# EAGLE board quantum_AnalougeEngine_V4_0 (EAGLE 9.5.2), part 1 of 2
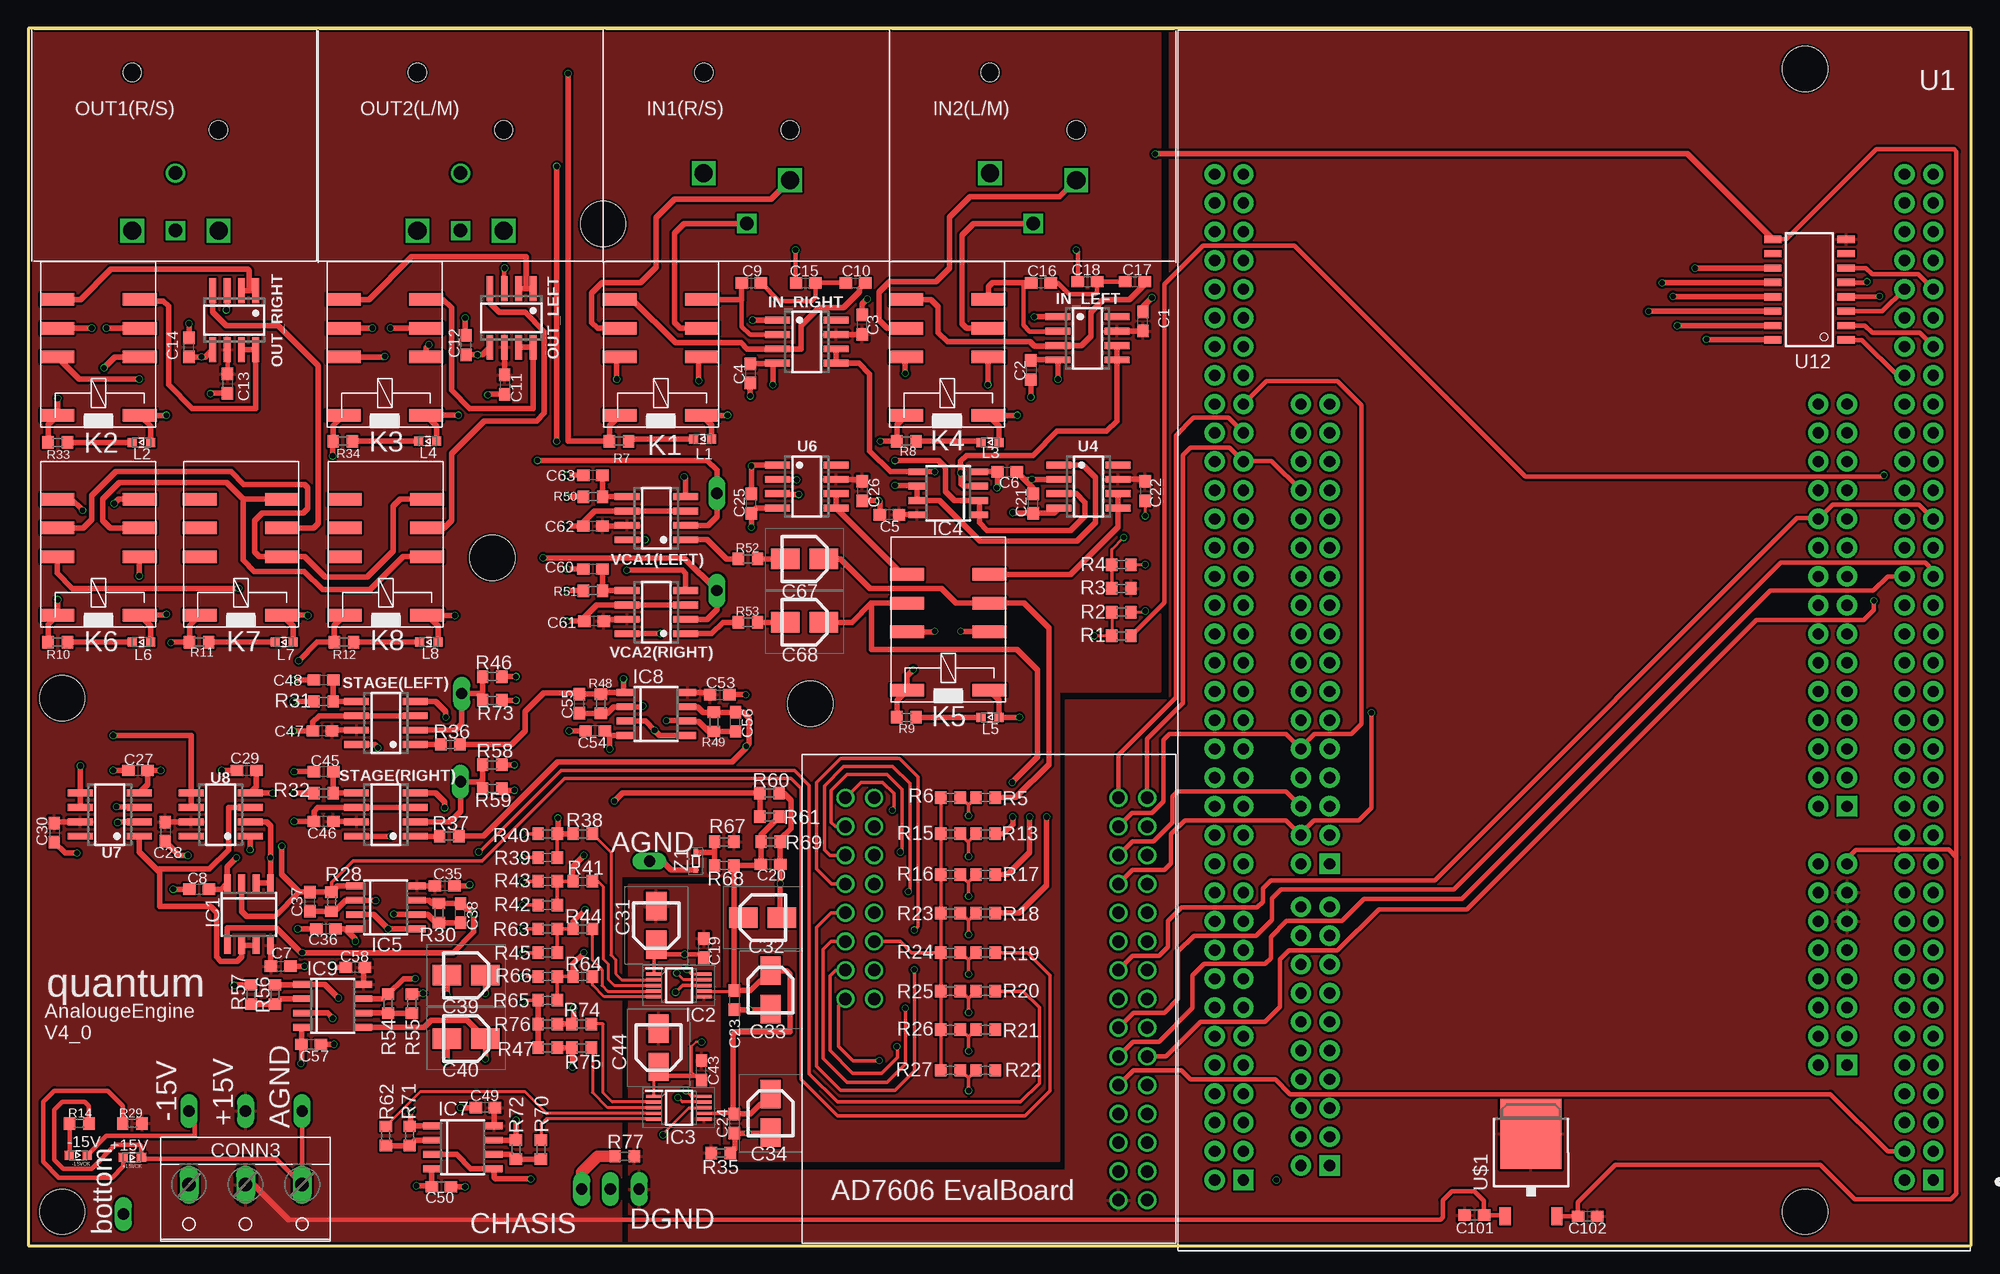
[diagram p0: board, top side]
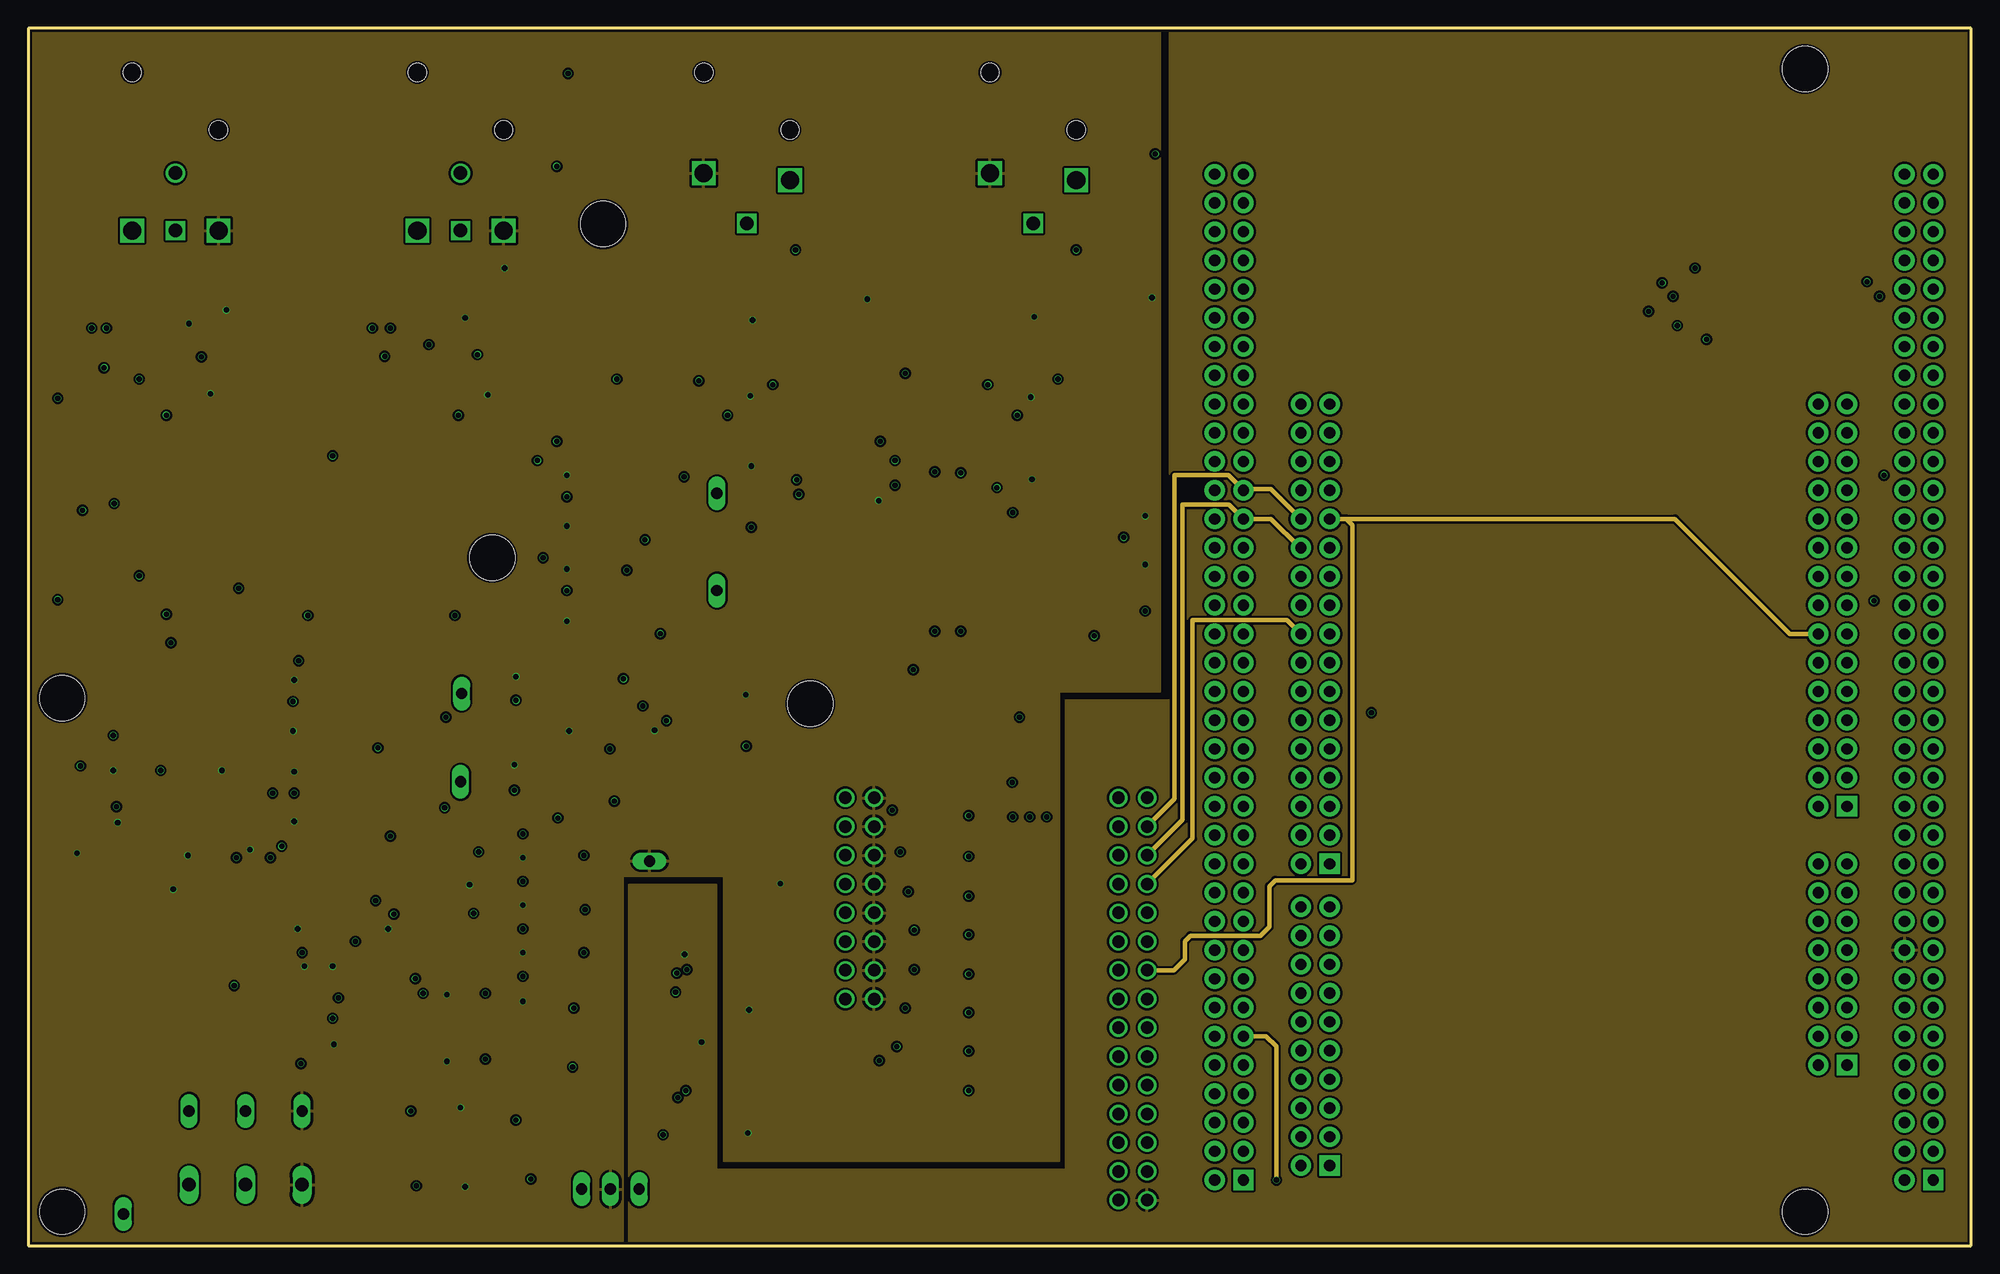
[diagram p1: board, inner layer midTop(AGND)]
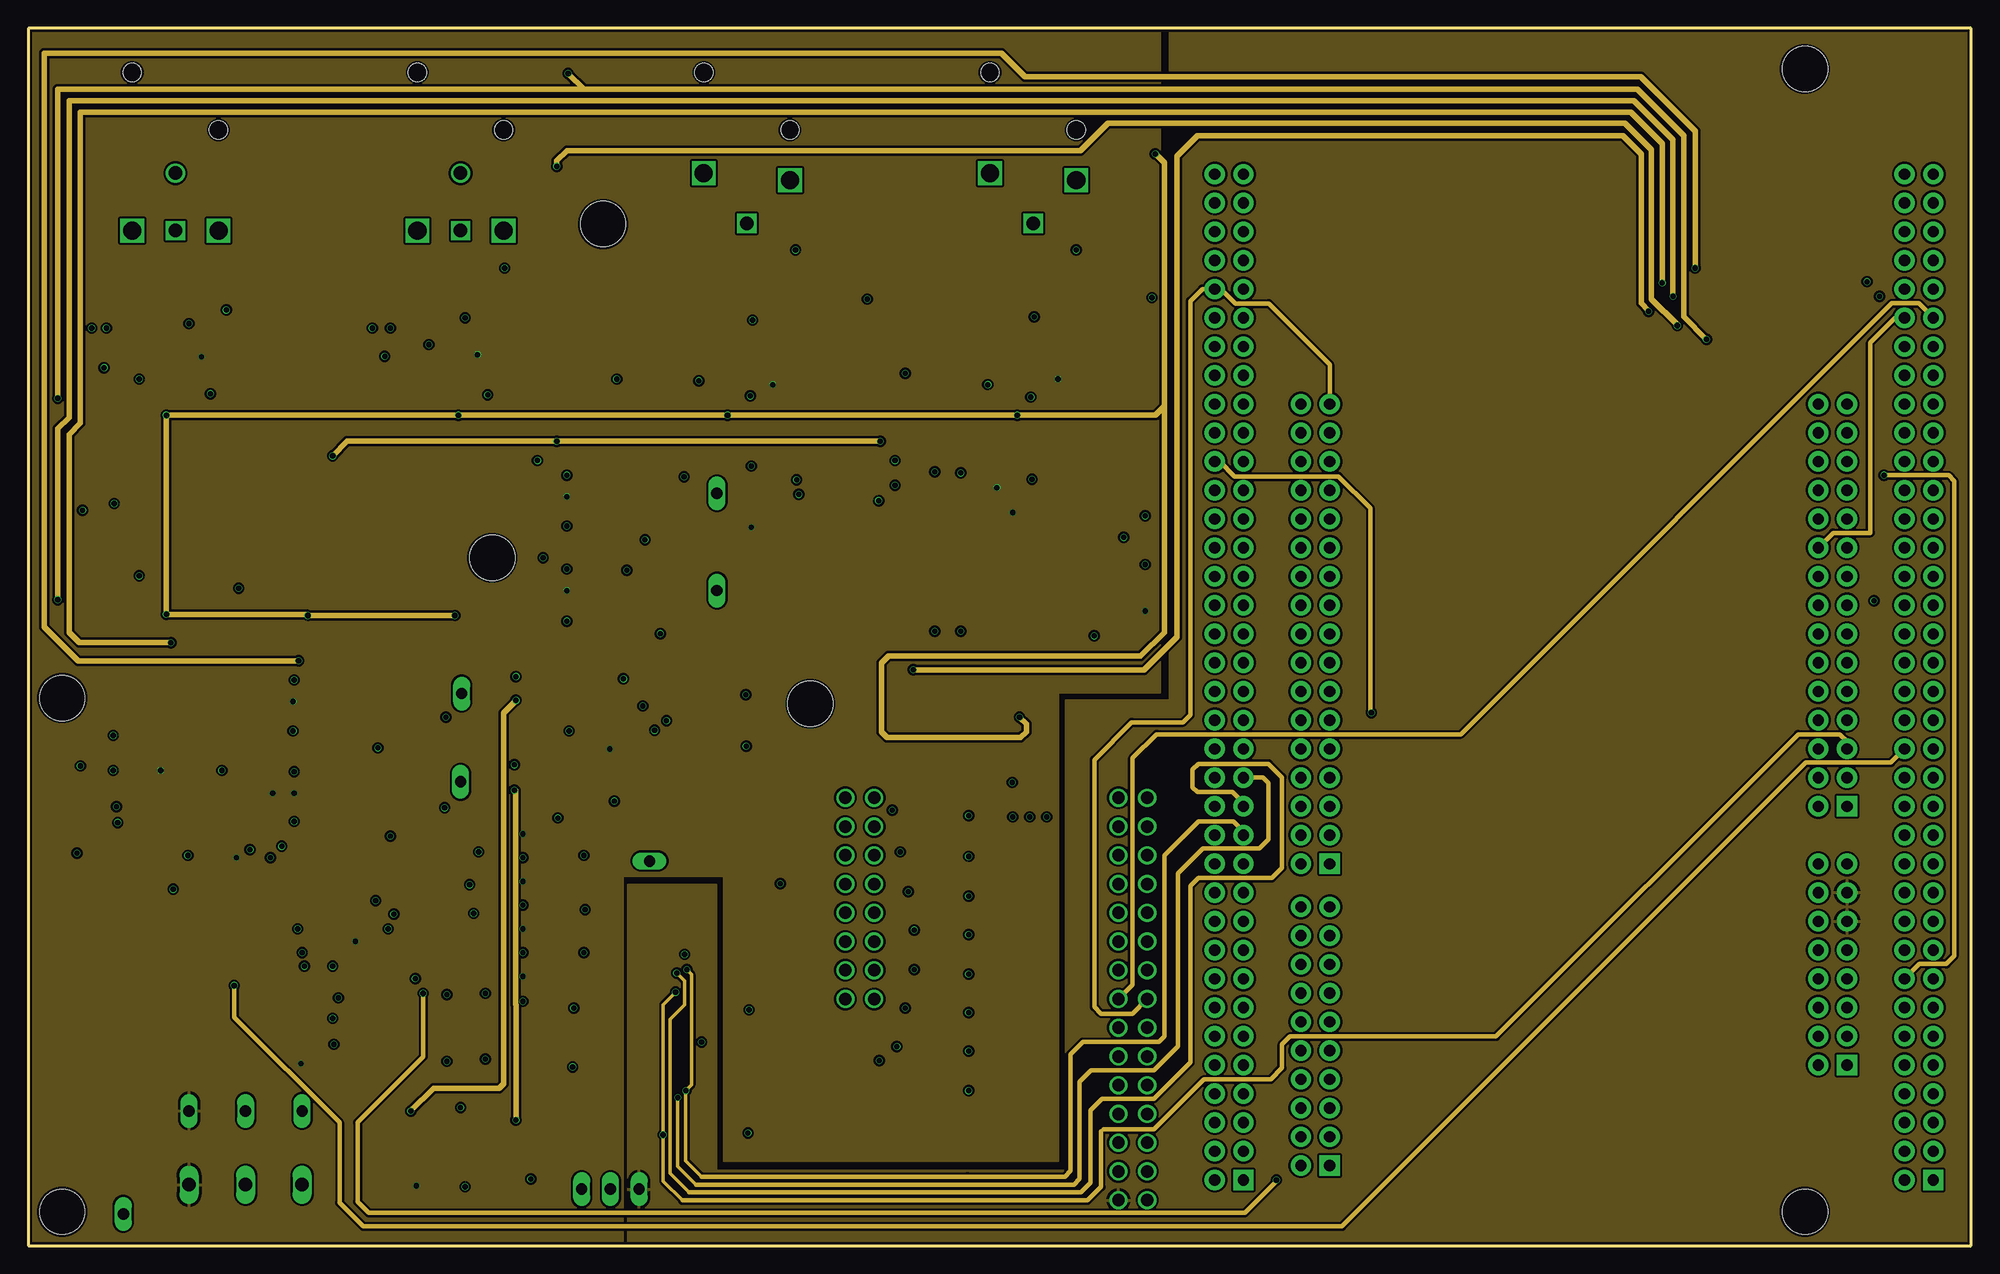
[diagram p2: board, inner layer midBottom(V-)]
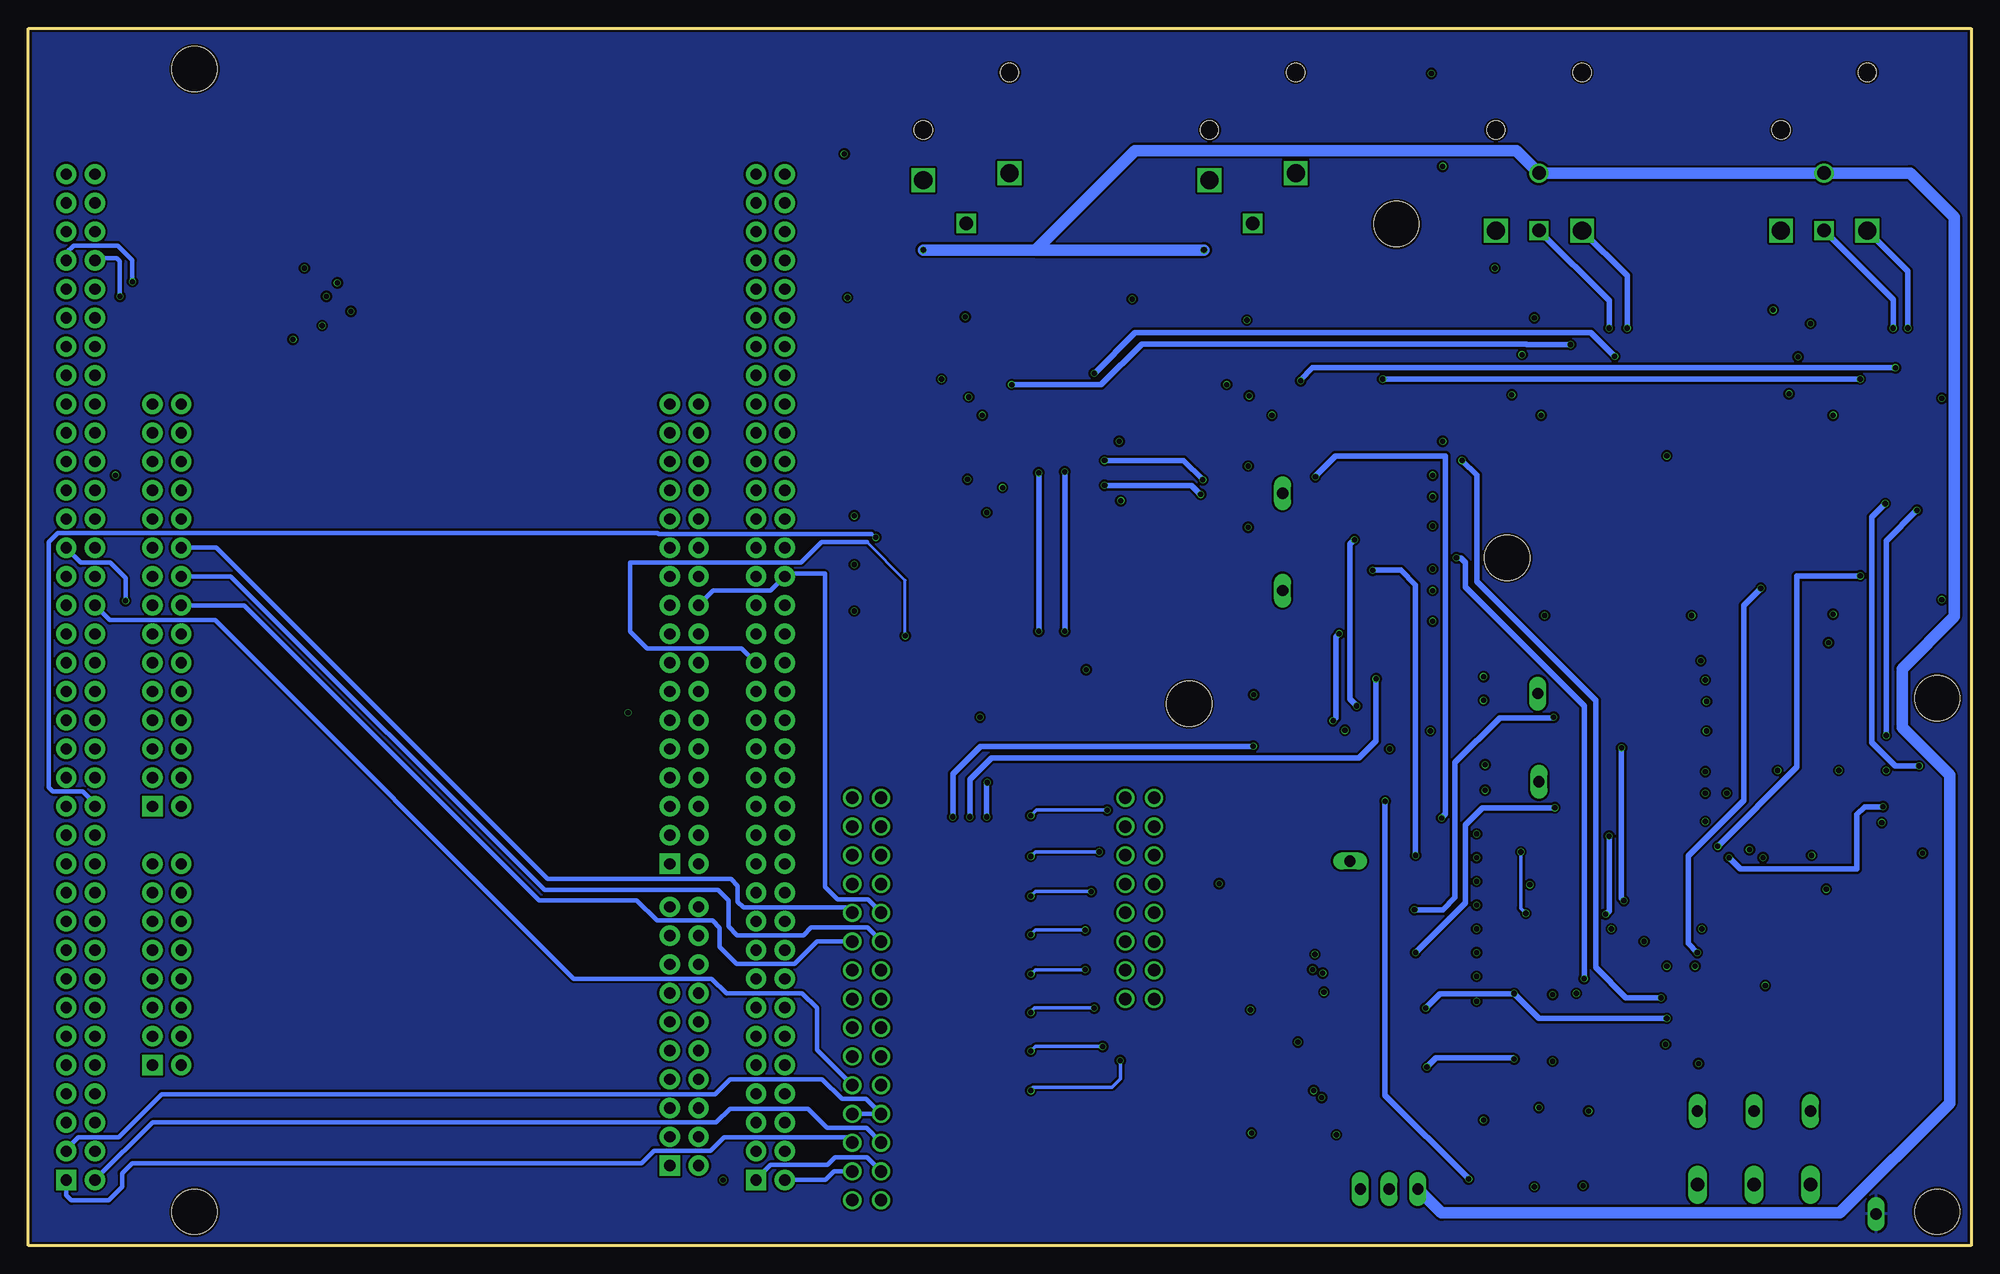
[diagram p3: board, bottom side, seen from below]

Size 171.7 x 107.6 mm. Coordinates in mm from the lower left corner, seen from the top.
Outline: 0,0 171.7,0 171.7,107.6 0,107.6 0,0
Copper layers (1*2+15*16): Top(V+) 0.018mm / dielectric 0.362mm / midTop(AGND) 0.035mm / dielectric 0.71mm / midBottom(V-) 0.035mm / dielectric 0.362mm / Bottom 0.018mm
Design rules "4layer": minimum track width 0.2mm, minimum drill 0.2mm, track to track 0.2mm, track to pad 0.1mm, pad to pad 0.1mm, via to via 0.1mm, smd to smd 0.1mm, copper to edge 0.2mm, drill to drill 0.21mm, minimum pad ring 0.25mm, minimum via ring 0.05mm, stop-mask expansion 0.01mm, vias tented up to drill 0mil, thermal gap 10mil
Holes 4 mm at 3,3 157,3 69.1,47.9 157,104 50.8,90.3 41,60.8 3,48.4

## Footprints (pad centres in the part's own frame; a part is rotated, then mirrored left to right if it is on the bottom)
WL-SMCW_0603 = smd 0.8 x 0.8: 1 -0.8,0; 2 0.8,0
C0603 = smd 1.1 x 1: 1 -0.85,0; 2 0.85,0
CAPAE400X550N = smd 2.5 x 1.8: 1 -1.7,0; 2 1.7,0
W237-103 = drill 1.194 long: 1 -5,-1.29; 2 0,-1.29; 3 5,-1.29
SOIC8 = smd 0.6 x 1.5: 1 -1.905,-2.75; 2 -0.635,-2.75; 3 0.635,-2.75; 4 1.905,-2.75; 5 1.905,2.75; 6 0.635,2.75; 7 -0.635,2.75; 8 -1.905,2.75
SOP50P490X110-10N = smd 1.4 x 0.3: 1 -2.2,1; 2 -2.2,0.5; 3 -2.2,0; 4 -2.2,-0.5; 5 -2.2,-1; 6 2.2,-1; 7 2.2,-0.5; 8 2.2,0; 9 2.2,0.5; 10 2.2,1
NEUTRIK_NC3FAH = drill 1.6 square: 1 -3.81,-12.7; 2 3.81,-13.335 | drill 1.2 square: 3 0,-17.15 | hole 1.6: -3.81,-3.81; 3.81,-8.89
SO08 = smd 0.6 x 2.2: 1 -1.905,-2.6; 2 -0.635,-2.6; 3 0.635,-2.6; 4 1.905,-2.6; 5 1.905,2.6; 6 0.635,2.6; 7 -0.635,2.6; 8 -1.905,2.6
351 = smd 1.11 x 3: 1 -2.623,-3.645; 2 -2.623,3.645; P1 5.096,-3.645; P2 5.096,3.645; Q1 2.556,-3.645; Q2 2.556,3.645; S1 7.636,-3.645; S2 7.636,3.645
NEUTRIK_NC3MAH = drill 1.6 square: 1 3.81,-17.78; 2 -3.81,-17.78 | drill 1.2 square: 3 0,-17.78 | drill 1.2: G 0,-12.7 | hole 1.6: -3.81,-3.8; 3.81,-8.89
R0603 = smd 1 x 1.1: 1 -0.85,0; 2 0.85,0
THT_PIN = drill 1 long: P$1 0,0
MODULE_NUCLEO-F429ZI = drill 1 pad 1.8 square: CN7_1 21.59,43.82; CN8_1 -24.13,34.93; CN9_1 -24.13,12.07; CN10_1 21.59,17.15; CN11_1 -31.75,45.09; CN12_1 29.21,45.09 | drill 1 pad 1.8: CN7_2 24.13,43.82; CN7_3 21.59,41.28; CN7_4 24.13,41.28; CN7_5 21.59,38.74; CN7_6 24.13,38.74; CN7_7 21.59,36.2; CN7_8 24.13,36.2; CN7_9 21.59,33.66; CN7_10 24.13,33.66; CN7_11 21.59,31.12; CN7_12 24.13,31.12; CN7_13 21.59,28.58; CN7_14 24.13,28.58; CN7_15 21.59,26.04; CN7_16 24.13,26.04; CN7_17 21.59,23.5; CN7_18 24.13,23.5; CN7_19 21.59,20.96; CN7_20 24.13,20.96; CN8_2 -21.59,34.93; CN8_3 -24.13,32.39; CN8_4 -21.59,32.39; CN8_5 -24.13,29.85; CN8_6 -21.59,29.85; CN8_7 -24.13,27.31; CN8_8 -21.59,27.31; CN8_9 -24.13,24.77; CN8_10 -21.59,24.77; CN8_11 -24.13,22.23; CN8_12 -21.59,22.23; CN8_13 -24.13,19.69; CN8_14 -21.59,19.69; CN8_15 -24.13,17.15; CN8_16 -21.59,17.15; CN9_2 -21.59,12.07; CN9_3 -24.13,9.53; CN9_4 -21.59,9.53; CN9_5 -24.13,6.99; CN9_6 -21.59,6.99; CN9_7 -24.13,4.45; CN9_8 -21.59,4.45; CN9_9 -24.13,1.91; CN9_10 -21.59,1.91; CN9_11 -24.13,-0.63; CN9_12 -21.59,-0.63; CN9_13 -24.13,-3.17; CN9_14 -21.59,-3.17; CN9_15 -24.13,-5.71; CN9_16 -21.59,-5.71; CN9_17 -24.13,-8.25; CN9_18 -21.59,-8.25; CN9_19 -24.13,-10.79; CN9_20 -21.59,-10.79; CN9_21 -24.13,-13.33; CN9_22 -21.59,-13.33; CN9_23 -24.13,-15.87; CN9_24 -21.59,-15.87; CN9_25 -24.13,-18.41; CN9_26 -21.59,-18.41; CN9_27 -24.13,-20.95; CN9_28 -21.59,-20.95; CN9_29 -24.13,-23.49; CN9_30 -21.59,-23.49; CN10_2 24.13,17.15; CN10_3 21.59,14.61; CN10_4 24.13,14.61; CN10_5 21.59,12.07; CN10_6 24.13,12.07; CN10_7 21.59,9.53; CN10_8 24.13,9.53; CN10_9 21.59,6.99; CN10_10 24.13,6.99; CN10_11 21.59,4.45; CN10_12 24.13,4.45; CN10_13 21.59,1.91; CN10_14 24.13,1.91; CN10_15 21.59,-0.63; CN10_16 24.13,-0.63; CN10_17 21.59,-3.17; CN10_18 24.13,-3.17; CN10_19 21.59,-5.71; CN10_20 24.13,-5.71; CN10_21 21.59,-8.25; CN10_22 24.13,-8.25; CN10_23 21.59,-10.79; CN10_24 24.13,-10.79; CN10_25 21.59,-13.33; CN10_26 24.13,-13.33; CN10_27 21.59,-15.87; CN10_28 24.13,-15.87; CN10_29 21.59,-18.41; CN10_30 24.13,-18.41; CN10_31 21.59,-20.95; CN10_32 24.13,-20.95; CN10_33 21.59,-23.49; CN10_34 24.13,-23.49; CN11_2 -29.21,45.09; CN11_3 -31.75,42.55; CN11_4 -29.21,42.55; CN11_5 -31.75,40.01; CN11_6 -29.21,40.01; CN11_7 -31.75,37.47; CN11_8 -29.21,37.47; CN11_9 -31.75,34.93; CN11_10 -29.21,34.93; CN11_11 -31.75,32.39; CN11_12 -29.21,32.39; CN11_13 -31.75,29.85; CN11_14 -29.21,29.85; CN11_15 -31.75,27.31; CN11_16 -29.21,27.31; CN11_17 -31.75,24.77; CN11_18 -29.21,24.77; CN11_19 -31.75,22.23; CN11_20 -29.21,22.23; CN11_21 -31.75,19.69; CN11_22 -29.21,19.69; CN11_23 -31.75,17.15; CN11_24 -29.21,17.15; CN11_25 -31.75,14.61; CN11_26 -29.21,14.61; CN11_27 -31.75,12.07; CN11_28 -29.21,12.07; CN11_29 -31.75,9.53; CN11_30 -29.21,9.53; CN11_31 -31.75,6.99; CN11_32 -29.21,6.99; CN11_33 -31.75,4.45; CN11_34 -29.21,4.45; CN11_35 -31.75,1.91; CN11_36 -29.21,1.91; CN11_37 -31.75,-0.63; CN11_38 -29.21,-0.63; CN11_39 -31.75,-3.17; CN11_40 -29.21,-3.17; CN11_41 -31.75,-5.71; CN11_42 -29.21,-5.71; CN11_43 -31.75,-8.25; CN11_44 -29.21,-8.25; CN11_45 -31.75,-10.79; CN11_46 -29.21,-10.79; CN11_47 -31.75,-13.33; CN11_48 -29.21,-13.33; CN11_49 -31.75,-15.87; CN11_50 -29.21,-15.87; CN11_51 -31.75,-18.41; CN11_52 -29.21,-18.41; CN11_53 -31.75,-20.95; CN11_54 -29.21,-20.95; CN11_55 -31.75,-23.49; CN11_56 -29.21,-23.49; CN11_57 -31.75,-26.03; CN11_58 -29.21,-26.03; CN11_59 -31.75,-28.57; CN11_60 -29.21,-28.57; CN11_61 -31.75,-31.11; CN11_62 -29.21,-31.11; CN11_63 -31.75,-33.65; CN11_64 -29.21,-33.65; CN11_65 -31.75,-36.19; CN11_66 -29.21,-36.19; CN11_67 -31.75,-38.73; CN11_68 -29.21,-38.73; CN11_69 -31.75,-41.27; CN11_70 -29.21,-41.27; CN11_71 -31.75,-43.81; CN11_72 -29.21,-43.81; CN12_2 31.75,45.09; CN12_3 29.21,42.55; CN12_4 31.75,42.55; CN12_5 29.21,40.01; CN12_6 31.75,40.01; CN12_7 29.21,37.47; CN12_8 31.75,37.47; CN12_9 29.21,34.93; CN12_10 31.75,34.93; CN12_11 29.21,32.39; CN12_12 31.75,32.39; CN12_13 29.21,29.85; CN12_14 31.75,29.85; CN12_15 29.21,27.31; CN12_16 31.75,27.31; CN12_17 29.21,24.77; CN12_18 31.75,24.77; CN12_19 29.21,22.23; CN12_20 31.75,22.23; CN12_21 29.21,19.69; CN12_22 31.75,19.69; CN12_23 29.21,17.15; CN12_24 31.75,17.15; CN12_25 29.21,14.61; CN12_26 31.75,14.61; CN12_27 29.21,12.07; CN12_28 31.75,12.07; CN12_29 29.21,9.53; CN12_30 31.75,9.53; CN12_31 29.21,6.99; CN12_32 31.75,6.99; CN12_33 29.21,4.45; CN12_34 31.75,4.45; CN12_35 29.21,1.91; CN12_36 31.75,1.91; CN12_37 29.21,-0.63; CN12_38 31.75,-0.63; CN12_39 29.21,-3.17; CN12_40 31.75,-3.17; CN12_41 29.21,-5.71; CN12_42 31.75,-5.71; CN12_43 29.21,-8.25; CN12_44 31.75,-8.25; CN12_45 29.21,-10.79; CN12_46 31.75,-10.79; CN12_47 29.21,-13.33; CN12_48 31.75,-13.33; CN12_49 29.21,-15.87; CN12_50 31.75,-15.87; CN12_51 29.21,-18.41; CN12_52 31.75,-18.41; CN12_53 29.21,-20.95; CN12_54 31.75,-20.95; CN12_55 29.21,-23.49; CN12_56 31.75,-23.49; CN12_57 29.21,-26.03; CN12_58 31.75,-26.03; CN12_59 29.21,-28.57; CN12_60 31.75,-28.57; CN12_61 29.21,-31.11; CN12_62 31.75,-31.11; CN12_63 29.21,-33.65; CN12_64 31.75,-33.65; CN12_65 29.21,-36.19; CN12_66 31.75,-36.19; CN12_67 29.21,-38.73; CN12_68 31.75,-38.73; CN12_69 29.21,-41.27; CN12_70 31.75,-41.27; CN12_71 29.21,-43.81; CN12_72 31.75,-43.81
SOIC16 = smd 1.524 x 0.635: 1 -3.24,4.445; 2 -3.24,3.175; 3 -3.24,1.905; 4 -3.24,0.635; 5 -3.24,-0.635; 6 -3.24,-1.905; 7 -3.24,-3.175; 8 -3.24,-4.445; 9 3.24,-4.445; 10 3.24,-3.175; 11 3.24,-1.905; 12 3.24,-0.635; 13 3.24,0.635; 14 3.24,1.905; 15 3.24,3.175; 16 3.24,4.445
TO252 = smd 1 x 1.6: 1 -2.28,-4.8; 3 2.28,-4.8 | smd 5.4 x 6.2: 2 0,2.5
AD7606_EVALBOARD = drill 1.1: +5V 30.48,-39.37; BUSY 27.94,-26.67; CS 30.48,-26.67; CVA 30.48,-31.75; CVB 27.94,-31.75; DB0 30.48,-21.59; DB1 27.94,-21.59; DB2 30.48,-19.05; DB3 27.94,-19.05; DB4 30.48,-16.51; DB5 27.94,-16.51; DB6 30.48,-13.97; DB7 27.94,-13.97; DB8 30.48,-11.43; DB9 27.94,-11.43; DB10 30.48,-8.89; DB11 27.94,-8.89; DB12 30.48,-6.35; DB13 27.94,-6.35; DB14 30.48,-3.81; DB15 27.94,-3.81; FRST 27.94,-24.13; G1 6.35,-3.81; G2 6.35,-6.35; G3 6.35,-8.89; G4 6.35,-11.43; G5 6.35,-13.97; G6 6.35,-16.51; G7 6.35,-19.05; G8 6.35,-21.59; GND 27.94,-39.37; OS0 30.48,-36.83; OS1 27.94,-36.83; OS2 30.48,-34.29; RANGE 27.94,-34.29; RD 27.94,-29.21; RST 30.48,-29.21; V1 3.81,-3.81; V2 3.81,-6.35; V3 3.81,-8.89; V4 3.81,-11.43; V5 3.81,-13.97; V6 3.81,-16.51; V7 3.81,-19.05; V8 3.81,-21.59; VIO 30.48,-24.13
SODFL1608X65N = smd 0.57 x 0.42: 1 -0.775,0; 2 0.775,0

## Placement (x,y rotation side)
+15VOK  SMD_LED_0603  [WL-SMCW_0603]  9.2,7.8 180 top
-15VOK  SMD_LED_0603  [WL-SMCW_0603]  4.4,8 180 top
C1  100nF  [C0603]  98.5,81.7 90 top
C2  100nF  [C0603]  88.6,77.4 270 top
C3  100nF  [C0603]  73.7,81.4 90 top
C4  100nF  [C0603]  63.8,77.1 270 top
C5  100nF  [C0603]  76.1,64.6 180 top
C6  100nF  [C0603]  86.5,68.4 0 top
C7  100nF  [C0603]  22.3,24.7 0 top
C8  100nF  [C0603]  15.1,31.5 180 top
C9  470 pF  [C0603]  63.9,85.1 0 top
C10  470 pF  [C0603]  73.1,85.1 0 top
C11  100nF  [C0603]  42.1,76.1 270 top
C12  100nF  [C0603]  38.7,79.6 90 top
C13  100nF  [C0603]  17.6,76.2 270 top
C14  100nF  [C0603]  14.2,79.4 90 top
C15  47 pF  [C0603]  68.7,85.1 0 top
C16  470 pF  [C0603]  89.5,85.1 0 top
C17  470 pF  [C0603]  97.8,85.2 0 top
C18  47 pF  [C0603]  93.6,85.2 0 top
C19  100nF  [C0603]  59.7,26.3 90 top
C20  100nF  [C0603]  65.6,33.7 0 top
C21  100nF  [C0603]  88.8,65.6 90 top
C22  100nF  [C0603]  98.7,66.7 270 top
C23  100nF  [C0603]  62.4,21.7 270 top
C24  100nF  [C0603]  62.4,10.8 270 top
C25  100nF  [C0603]  63.9,65.6 90 top
C26  100nF  [C0603]  73.7,66.7 270 top
C27  100nF  [C0603]  9.7,42 180 top
C28  100nF  [C0603]  12.1,36.6 270 top
C29  100nF  [C0603]  19.3,42 180 top
C30  100nF  [C0603]  2.3,36.5 270 top
C31  10 µF  [CAPAE400X550N]  55.5,28.3 90 top
C32  10 µF  [CAPAE400X550N]  64.9,29 0 top
C33  10 µF  [CAPAE400X550N]  65.6,22.6 270 top
C34  10 µF  [CAPAE400X550N]  65.6,11.7 270 top
C35  100nF  [C0603]  36.8,31.8 0 top
C36  100nF  [C0603]  26.3,28 180 top
C37  22pF  [C0603]  24.9,30.4 90 top
C38  22pF  [C0603]  38.2,29.4 90 top
C39  10 µF  [CAPAE400X550N]  38.7,23.9 180 top
C40  10 µF  [CAPAE400X550N]  38.7,18.3 180 top
C43  100nF  [C0603]  59.5,15.5 90 top
C44  10 µF  [CAPAE400X550N]  55.7,17.5 90 top
C45  100nF  [C0603]  26.1,41.9 180 top
C46  100nF  [C0603]  26.1,37.5 180 top
C47  100nF  [C0603]  26,45.5 180 top
C48  100nF  [C0603]  26.1,50 180 top
C49  100nF  [C0603]  40.4,12.2 180 top
C50  100nF  [C0603]  36.5,5.2 0 top
C53  100nF  [C0603]  61.1,48.7 0 top
C54  100nF  [C0603]  50.1,45.5 180 top
C55  22pF  [C0603]  48.7,47.9 90 top
C56  22pF  [C0603]  62.5,46.3 90 top
C57  100nF  [C0603]  25,17.8 0 top
C58  100nF  [C0603]  28.9,24.6 180 top
C60  100nF  [C0603]  49.9,59.8 180 top
C61  100nF  [C0603]  50,55.2 180 top
C62  100nF  [C0603]  49.9,63.6 180 top
C63  100nF  [C0603]  49.9,68.1 180 top
C67  47µF  [CAPAE400X550N]  68.6,60.7 180 top
C68  47µF  [CAPAE400X550N]  68.6,55.1 180 top
C101  [C0603]  127.8,2.7 180 top
C102  [C0603]  137.8,2.6 0 top
CONN3  [W237-103]  19.2,4.1 180 top
IC1  OP275  [SOIC8]  19.5,29.3 180 top
IC2  DAC084S085CIMM_NOPB  [SOP50P490X110-10N]  57.5,23 0 top
IC3  DAC084S085CIMM_NOPB  [SOP50P490X110-10N]  57.5,12.2 0 top
IC4  OP275  [SOIC8]  81.3,66.5 90 top
IC5  OP275  [SOIC8]  31.6,29.9 270 top
IC7  TL072  [SOIC8]  38.4,8.7 270 top
IC8  OP275  [SOIC8]  55.5,47 270 top
IC9  TL072  [SOIC8]  26.9,21.2 270 top
IN1(R/S)  NEUTRIK_NC3FAH  [NEUTRIK_NC3FAH]  63.5,107.5 0 top
IN2(L/M)  NEUTRIK_NC3FAH  [NEUTRIK_NC3FAH]  88.8,107.5 0 top
IN_LEFT  1240  [SO08]  93.6,80.2 270 top
IN_RIGHT  1240  [SO08]  68.8,79.9 270 top
K1  K1  [351]  55.9,76 90 top
K2  K2  [351]  6.2,76 90 top
K3  K3  [351]  31.5,76 90 top
K4  K4  [351]  81.2,76 90 top
K5  RELAY_EE2-5NU  [351]  81.3,51.7 90 top
K6  RELAY_EE2-5NU  [351]  6.2,58.35 90 top
K7  RELAY_EE2-5NU  [351]  18.8,58.35 90 top
K8  RELAY_EE2-5NU  [351]  31.6,58.35 90 top
L1  SMD_LED_0603  [WL-SMCW_0603]  59.6,71.3 0 top
L2  SMD_LED_0603  [WL-SMCW_0603]  10,71 0 top
L3  SMD_LED_0603  [WL-SMCW_0603]  85,71 0 top
L4  SMD_LED_0603  [WL-SMCW_0603]  35.3,71.1 0 top
L5  SMD_LED_0603  [WL-SMCW_0603]  85,46.7 0 top
L6  SMD_LED_0603  [WL-SMCW_0603]  10,53.35 0 top
L7  SMD_LED_0603  [WL-SMCW_0603]  22.6,53.35 0 top
L8  SMD_LED_0603  [WL-SMCW_0603]  35.4,53.35 0 top
OUT1(R/S)  NEUTRIK_NC3MAH  [NEUTRIK_NC3MAH]  13,107.5 0 top
OUT2(L/M)  NEUTRIK_NC3MAH  [NEUTRIK_NC3MAH]  38.2,107.5 0 top
OUT_LEFT  1646  [SO08]  42.7,82 180 top
OUT_RIGHT  1646  [SO08]  18.2,81.8 180 top
R1  10k  [R0603]  96.6,53.9 0 top
R2  100k  [R0603]  96.6,56 180 top
R3  100k  [R0603]  96.6,58.1 0 top
R4  10k  [R0603]  96.6,60.2 180 top
R5  10k  [R0603]  84.6,39.6 180 top
R6  10k  [R0603]  81.5,39.6 0 top
R7  500R  [R0603]  52.2,71.1 0 top
R8  500R  [R0603]  77.6,71.1 0 top
R9  500R  [R0603]  77.6,46.7 0 top
R10  500R  [R0603]  2.6,53.35 0 top
R11  500R  [R0603]  15.1,53.35 0 top
R12  500R  [R0603]  27.9,53.35 0 top
R13  10k  [R0603]  84.6,36.4 180 top
R14  220R  [R0603]  4.5,10.8 0 top
R15  10k  [R0603]  81.5,36.4 0 top
R16  10k  [R0603]  81.5,32.8 0 top
R17  10k  [R0603]  84.6,32.8 180 top
R18  10k  [R0603]  84.6,29.4 180 top
R19  10k  [R0603]  84.6,25.9 180 top
R20  10k  [R0603]  84.6,22.5 180 top
R21  10k  [R0603]  84.6,19.1 180 top
R22  10k  [R0603]  84.6,15.5 180 top
R23  10k  [R0603]  81.5,29.4 0 top
R24  10k  [R0603]  81.5,25.9 0 top
R25  10k  [R0603]  81.5,22.5 0 top
R26  10k  [R0603]  81.5,19.1 0 top
R27  10k  [R0603]  81.5,15.5 0 top
R28  20k  [R0603]  26.8,30.4 90 top
R29  220R  [R0603]  9.2,10.8 0 top
R30  20k  [R0603]  36.3,29.4 90 top
R31  5k1  [R0603]  26.1,48.1 0 top
R32  5k1  [R0603]  26.1,40 0 top
R33  500R  [R0603]  2.6,71 0 top
R34  500R  [R0603]  27.8,71.1 0 top
R35  0R  [R0603]  61.2,8.2 180 top
R36  20k  [R0603]  37.3,44.3 180 top
R37  20k  [R0603]  37.2,36.2 180 top
R38  51k  [R0603]  49,36.4 0 top
R39  51R  [R0603]  45.9,34.3 0 top
R40  90k9  [R0603]  45.9,36.4 0 top
R41  51k  [R0603]  49,32.2 0 top
R42  51R  [R0603]  45.9,30.1 0 top
R43  90k9  [R0603]  45.9,32.2 0 top
R44  51k  [R0603]  49,28 0 top
R45  51R  [R0603]  45.9,25.9 0 top
R46  10k  [R0603]  41,50.3 180 top
R47  1k8  [R0603]  45.9,17.5 0 top
R48  20k  [R0603]  50.6,47.9 90 top
R49  20k  [R0603]  60.6,46.3 90 top
R50  5k1  [R0603]  49.9,66.2 0 top
R51  5k1  [R0603]  49.9,57.9 0 top
R52  20k  [R0603]  63.6,60.7 180 top
R53  20k  [R0603]  63.6,55.1 180 top
R54  10k  [R0603]  31.8,21.4 90 top
R55  10k  [R0603]  33.9,21.4 270 top
R56  10k  [R0603]  21.8,22.2 90 top
R57  10k  [R0603]  19.7,22.2 270 top
R58  10k  [R0603]  41,42.5 180 top
R59  56k  [R0603]  41,40.4 0 top
R60  10k  [R0603]  65.5,40 180 top
R61  10k  [R0603]  65.5,37.9 0 top
R62  10k  [R0603]  31.6,9.7 270 top
R63  90k9  [R0603]  45.9,28 0 top
R64  51k  [R0603]  49,23.8 0 top
R65  51R  [R0603]  45.9,21.7 0 top
R66  90k9  [R0603]  45.9,23.8 0 top
R67  10k  [R0603]  61.5,35.7 0 top
R68  10k  [R0603]  61.5,33.6 180 top
R69  10k  [R0603]  65.6,35.7 180 top
R70  10k  [R0603]  45.3,8.5 270 top
R71  10k  [R0603]  33.7,9.7 90 top
R72  10k  [R0603]  43.1,8.5 90 top
R73  10k  [R0603]  41,48.2 0 top
R74  10k  [R0603]  48.9,19.6 180 top
R75  10k  [R0603]  48.9,17.5 180 top
R76  1k8  [R0603]  45.9,19.6 0 top
R77  0R  [R0603]  52.7,7.9 0 top
STAGE(LEFT)  THAT2181S  [SO08]  31.6,46.2 90 top
STAGE(RIGHT)  THAT2181S  [SO08]  31.6,38.1 90 top
TP01  TPTHT  [THT_PIN]  38.2,41 90 top
TP02  TPTHT  [THT_PIN]  38.3,48.8 90 top
TP03  TPTHT  [THT_PIN]  48.9,5 90 top
TP04  TPTHT  [THT_PIN]  24.2,11.9 90 top
TP05  TPTHT  [THT_PIN]  53.98,5 90 top
TP06  TPTHT  [THT_PIN]  8.4,2.8 90 top
TP09  TPTHT  [THT_PIN]  19.2,11.9 270 top
TP16  TPTHT  [THT_PIN]  54.9,34 0 top
TP18  TPTHT  [THT_PIN]  51.44,5 90 top
TP23  TPTHT  [THT_PIN]  14.2,11.9 90 top
TP36  TPTHT  [THT_PIN]  60.85,57.9 90 top
TP37  TPTHT  [THT_PIN]  60.85,66.5 90 top
U1  NUCLEO-F429ZI  [MODULE_NUCLEO-F429ZI]  136.6,50.9 180 top
U4  THAT1240  [SO08]  93.7,67.1 270 top
U6  THAT1240  [SO08]  68.8,67.1 270 top
U7  THAT1240  [SO08]  7.2,38.1 90 top
U8  THAT1240  [SO08]  17,38.1 90 top
U12  ULN2003  [SOIC16]  157.4,84.5 180 top
U$1  7812  [TO252]  132.8,7.4 0 top
U$4  AD7606_EVALBOARD  [AD7606_EVALBOARD]  68.4,43.4 0 top
VCA1(LEFT)  THAT2181S  [SO08]  55.5,64.3 90 top
VCA2(RIGHT)  THAT2181S  [SO08]  55.5,56 90 top
Z1  BZT52C2V0T-7  [SODFL1608X65N]  59,34 270 top

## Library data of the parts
+15VOK -15VOK C1-C40 C43-C50 C53-C58 C60-C63 C67 C68 C101 C102 IC1 IC4 IC5 IC7-IC9 IN1(R/S) IN2(L/M) L1-L8 OUT1(R/S) OUT2(L/M) R2 R4 R6 R9-R12 R14-R16 R23-R77 TP01-TP06 TP09 TP16 TP18 TP23 TP36 TP37 U12 U$1 U$4 = C_Sager_Bibliothek
CONN3 = C_Sager_Bibliothek; MPN: 237-103; OC_FARNELL: unknown; OC_NEWARK: 18M7116
IC2 IC3 = SPI; DESCRIPTION: 8-Bit Micro Power QUAD Digital-to-Analog Converter with Rail-to-Rail Output; HEIGHT: 1.1mm; MANUFACTURER_NAME: Texas Instruments; MANUFACTURER_PART_NUMBER: DAC084S085CIMM/NOPB; MOUSER_PART_NUMBER: 926-DAC084S085CIMMNO; MOUSER_PRICE-STOCK: https://www.mouser.com/Search/Refine.aspx?Keyword=926-DAC084S085CIMMNO
IN_LEFT IN_RIGHT OUT_LEFT OUT_RIGHT STAGE(LEFT) STAGE(RIGHT) U4 U6-U8 VCA1(LEFT) VCA2(RIGHT) = THAT_Library
K1-K8 = C_Sager_Bibliothek; OC_FARNELL: unknown; OC_NEWARK: unknown
R1 R3 R5 R7 R8 R13 R17-R22 = C_Sager_Bibliothek; SPICEPREFIX: R
U1 = STM32_144; AVAILABILITY: Unavailable; DESCRIPTION: STM32 Nucleo-144 development board with STM32F429ZIT6 MCU, supports Arduino, ST Zio and Morpho; MF: STMicroelectronics; MP: NUCLEO-F429ZI; PACKAGE: None; PRICE: None
Z1 = C_Sager_Bibliothek; DESCRIPTION: Diodes Inc BZT52C2V0T-7 Zener Diode, 2.4V 5% 300 mW SMT 2-Pin SOD-523; HEIGHT: 0.65mm; MANUFACTURER_NAME: Diodes Inc.; MANUFACTURER_PART_NUMBER: BZT52C2V0T-7; MOUSER_PART_NUMBER: 621-BZT52C2V0T-7; MOUSER_PRICE-STOCK: https://www.mouser.com/Search/Refine.aspx?Keyword=621-BZT52C2V0T-7

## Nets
0,5V_DAC: IC7.3 IC7.5 R60.2 R61.1
1V_DAC: C20.1 C23.1 C24.1 C32.1 C33.1 C34.1 IC2.7 IC3.7 R61.2 R68.1 R69.2
2V_DAC_REF: R67.1 R68.2 Z1.1
+3V3_STM32: R1.2 U1.CN11_16
+5V_STM32: C19.1 C31.1 C43.1 C44.1 IC2.1 IC3.1 U1.CN11_18 U$4.+5V
+12V: C102.1 K1.1 K2.1 K3.1 K4.1 K5.1 K6.1 K7.1 K8.1 L1.2 L2.2 L3.2 L4.2 L5.2 L6.2 L7.2 L8.2 U1.CN8_15 U12.9 U$1.3
.: IC7.7 R59.2 R72.2
...: IC7.1 R71.2 R73.2
ADC1-IN0: R3.1 R4.2 U1.CN11_28
ADC1-IN3: R1.1 R2.2 U1.CN12_37
ADC1-IN6: U1.CN12_13
ADC2-IN9: U1.CN12_24
ADC2-IN10: U1.CN11_38
ADC2-IN12: U1.CN11_35
ADC3-IN13: U1.CN11_37
ADC3-IN14: U1.CN12_38
ADC3-IN15: U1.CN12_36
AGND: +15VOK.1 C1.2 C2.2 C3.2 C4.2 C5.2 C6.2 C7.2 C8.2 C11.2 C12.2 C13.2 C14.2 C20.2 C21.2 C22.2 C23.2 C24.2 C25.2 C26.2 C27.2 C28.2 C29.2 C30.2 C32.2 C33.2 C34.2 C35.2 C36.2 C39.2 C40.2 C45.2 C46.2 C47.2 C48.2 C49.2 C50.2 C53.2 C54.2 C57.2 C58.2 C60.2 C61.2 C62.2 C63.2 CONN3.1 IC5.3 IC5.5 IC8.3 IC8.5 IN1(R/S).1 IN2(L/M).1 IN_LEFT.1 IN_RIGHT.1 OUT1(R/S).1 OUT2(L/M).1 OUT_LEFT.3 OUT_RIGHT.3 R4.1 R6.1 R14.2 R15.1 R16.1 R23.1 R24.1 R25.1 R26.1 R27.1 R35.1 R39.1 R42.1 R45.1 R46.1 R47.1 R58.1 R60.1 R65.1 R69.1 R76.1 STAGE(LEFT).3 STAGE(LEFT).6 STAGE(RIGHT).3 STAGE(RIGHT).6 TP04.P$1 TP16.P$1 TP18.P$1 U4.2 U6.1 U7.2 U8.1 U$4.G1 U$4.G2 U$4.G3 U$4.G4 U$4.G5 U$4.G6 U$4.G7 U$4.G8 VCA1(LEFT).3 VCA1(LEFT).6 VCA2(RIGHT).3 VCA2(RIGHT).6 Z1.2
BOTTOM: TP06.P$1
BUSY: U1.CN11_44 U$4.BUSY
CHASIS: C15.1 C18.1 OUT1(R/S).G OUT2(L/M).G R77.1 TP03.P$1
CS: U1.CN11_45 U$4.CS
CS_DAC1: IC2.9 U1.CN12_27
CS_DAC2: IC3.9 U1.CN12_29
CV_A_B: U1.CN11_3 U$4.CVA U$4.CVB
DAC2_OUT1(OFFSET_VCA1): C39.1 IC9.3 R74.2 R76.2
DAC2_OUT2(OFFSET_VCA2): C40.1 IC9.5 R47.2 R75.2
DAC2_OUT3: IC3.4 R62.1
DAC2_OUT4: IC3.5 R70.1
DAC_OUT1: R57.1 U1.CN11_32
DAC_OUT2: R55.1 U1.CN12_11
DB0: U1.CN10_33 U1.CN12_64 U$4.DB0
DB1: U1.CN11_61 U$4.DB1
DB2: U1.CN9_14 U1.CN10_25 U$4.DB2
DB3: U1.CN9_22 U1.CN11_47 U$4.DB3
DB4: U1.CN9_16 U$4.DB4
DB5: U1.CN9_18 U$4.DB5
DB6: U1.CN9_20 U1.CN11_62 U$4.DB6
DB7: U1.CN10_20 U1.CN12_44 U$4.DB7
DB8: U1.CN10_18 U$4.DB8
DB9: U1.CN10_4 U1.CN12_52 U$4.DB9
DB10: U1.CN10_24 U1.CN12_47 U$4.DB10
DB11: U1.CN10_6 U$4.DB11
DB12: U1.CN10_26 U1.CN12_49 U$4.DB12
DB13: U1.CN10_10 U1.CN12_55 U$4.DB13
DB14: U1.CN10_28 U1.CN12_51 U$4.DB14
DB15: U1.CN12_53 U$4.DB15
DGND: C19.2 C31.2 C43.2 C44.2 C101.2 C102.2 IC2.6 IC3.6 R35.2 R77.2 TP05.P$1 U1.CN8_11 U1.CN8_13 U12.8 U$1.2 U$4.GND
DIN_DAC: IC2.8 IC3.8 U1.CN9_5
E+_OUT_STAGE_LEFT: R46.2 R73.1 STAGE(LEFT).2 TP02.P$1
E+_OUT_STAGE_RIGHT: R58.2 R59.1 STAGE(RIGHT).2 TP01.P$1
EC+_VCA1(LFT): IC9.1 R56.2 TP37.P$1 VCA1(LEFT).2
EC+_VCA2(RIGHT): IC9.7 R54.2 TP36.P$1 VCA2(RIGHT).2
FRST: U1.CN11_43 U$4.FRST
L: IC4.3 IN_LEFT.5 IN_LEFT.6 K5.Q1
L/M_IN(VCA1_IN): C67.1 K5.P1 R5.1
L/M_OUT(OUT_STAGE_LEFT): C37.2 IC1.3 IC5.1 K6.Q1 R19.1 R28.2
L/M_OUT(VCA1_OUT): C55.2 IC8.1 R17.1 R36.1 R48.2
L/M_OUT+: K3.S1 OUT_LEFT.7 OUT_LEFT.8
L/M_OUT-: K3.S2 OUT_LEFT.1 OUT_LEFT.2
M: K5.S1 U4.5 U4.6
M1: K6.S1 U7.5 U7.6
N$1: C9.1 IN_RIGHT.2 K1.S1
N$2: C10.2 IN_RIGHT.3 K1.S2
N$3: C9.2 C10.1 C15.2
N$4: R5.2 R6.2 U$4.V1
N$5: K6.P1 K7.S1 K8.Q1
N$6: R13.2 R15.2 U$4.V2
N$7: C17.2 IN_LEFT.3 K4.S2
N$8: K1.Q1 K2.Q1
N$9: C16.2 C17.1 C18.2
N$10: R16.2 R17.2 U$4.V3
N$11: K1.Q2 K2.Q2
N$12: R18.2 R23.2 U$4.V4
N$13: C16.1 IN_LEFT.2 K4.S1
N$14: L1.1 R7.2
N$15: K3.P1 OUT2(L/M).3
N$16: L3.1 R8.2
N$17: K3.P2 OUT2(L/M).2
N$18: IC4.1 IC4.2 U4.3 U6.2
N$19: K6.P2 K7.Q1 K8.S1
N$20: R19.2 R24.2 U$4.V5
N$21: IN1(R/S).2 K1.P2
N$22: IN1(R/S).3 K1.P1
N$23: K2.P2 OUT1(R/S).2
N$24: K2.P1 OUT1(R/S).3
N$25: IN2(L/M).3 K4.P1
N$26: L8.1 R12.2
N$27: IN2(L/M).2 K4.P2
N$28: K3.Q1 K4.Q1
N$29: L7.1 R11.2
N$30: L6.1 R10.2
N$31: K3.Q2 K4.Q2
N$32: L5.1 R9.2
N$33: IC4.6 IC4.7 U4.1 U6.3
N$34: R20.2 R25.2 U$4.V6
N$35: R21.2 R26.2 U$4.V7
N$36: R22.2 R27.2 U$4.V8
N$37: U1.CN8_7
N$43: IC1.6 IC1.7 U7.1 U8.3
N$45: IC1.1 IC1.2 U7.3 U8.2
N$46: R21.1
N$47: R22.1
N$48: C37.1 IC5.2 R28.1 STAGE(LEFT).8
N$49: L2.1 R33.2
N$50: -15VOK.2 R14.1
N$51: L4.1 R34.2
N$52: +15VOK.2 R29.1
N$53: C38.1 IC5.6 R30.1 STAGE(RIGHT).8
N$54: C45.1 R32.2 STAGE(RIGHT).5
N$55: R36.2 STAGE(LEFT).1
N$56: IC2.2 R38.2
N$57: IC2.3 R41.2
N$58: IC2.4 R44.2
N$59: IC2.5 R64.2
N$60: IC3.2 R74.1
N$61: IC3.3 R75.1
N$63: IC9.2 R56.1 R57.2
N$64: C55.1 IC8.2 R48.1 VCA1(LEFT).8
N$65: R52.2 VCA1(LEFT).1
N$68: R37.2 STAGE(RIGHT).1
N$71: C67.2 R52.1
N$72: IC7.2 R62.2 R71.1
N$73: C48.1 R31.2 STAGE(LEFT).5
N$74: IC7.6 R70.2 R72.1
N$75: C56.1 IC8.6 R49.1 VCA2(RIGHT).8
N$77: C60.1 R51.2 VCA2(RIGHT).5
N$78: C68.2 R53.1
N$79: R53.2 VCA2(RIGHT).1
N$80: C63.1 R50.2 VCA1(LEFT).5
N$81: IC9.6 R54.1 R55.2
OS0: U1.CN12_2 U$4.OS0
OS1: U1.CN12_1 U$4.OS1
OS2: U1.CN11_1 U$4.OS2
OUT1_DRIVER: K1.2 K2.2 R7.1 R33.1 U12.16
OUT2_DRIVER: K3.2 K4.2 R8.1 R34.1 U12.15
OUT3_DRIVER: K5.2 R9.1 U12.14
OUT4_DRIVER: K6.2 R10.1 U12.13
OUT5_DRIVER: K7.2 R11.1 U12.12
OUT6_DRIVER: K8.2 R12.1 U12.11
OUT_L/M: K8.P1 OUT_LEFT.4
OUT_R/S: K7.P1 OUT_RIGHT.4
R: IC4.5 IN_RIGHT.5 IN_RIGHT.6 K5.Q2
R/S_IN(VCA2_IN): C68.1 K5.P2 R13.1
R/S_OUT(OUT_STAGE_RIGHT): C38.2 IC1.5 IC5.7 K6.Q2 R20.1 R30.2
R/S_OUT(VCA2_OUT): C56.2 IC8.7 R18.1 R37.1 R49.2
R/S_OUT+: K2.S1 OUT_RIGHT.7 OUT_RIGHT.8
R/S_OUT-: K2.S2 OUT_RIGHT.1 OUT_RIGHT.2
RANGE: U1.CN11_2 U$4.RANGE
RD: U1.CN11_4 U$4.RD
RELAIS1: U1.CN11_58 U12.1
RELAIS2: U1.CN11_59 U12.2
RELAIS3: U1.CN11_64 U12.3
RELAIS4: U1.CN11_66 U12.4
RELAIS5: U1.CN11_65 U12.5
RELAIS6: U1.CN11_63 U12.6
RESET: U1.CN11_42 U$4.RST
S: K5.S2 U6.5 U6.6
S1: K6.S2 U8.5 U8.6
SCLK_DAC: IC2.10 IC3.10 U1.CN12_25
SYM1: R38.1 R39.2 R40.2 VCA1(LEFT).4
SYM2: R41.1 R42.2 R43.2 VCA2(RIGHT).4
SYM3: R44.1 R45.2 R63.2 STAGE(LEFT).4
SYM4: R64.1 R65.2 R66.2 STAGE(RIGHT).4
USART6_TX: U1.CN12_4
USRAT6_RX: U1.CN12_19
V+: C1.1 C3.1 C5.1 C7.1 C11.1 C13.1 C22.1 C26.1 C28.1 C30.1 C35.1 C46.1 C47.1 C49.1 C53.1 C58.1 C61.1 C62.1 C101.1 CONN3.2 IC1.8 IC4.8 IC5.8 IC7.8 IC8.8 IC9.8 IN_LEFT.7 IN_RIGHT.7 OUT_LEFT.6 OUT_RIGHT.6 R3.2 R29.2 R67.2 STAGE(LEFT).7 STAGE(RIGHT).7 TP09.P$1 U4.7 U6.7 U7.7 U8.7 U$1.1 VCA1(LEFT).7 VCA2(RIGHT).7
V-: -15VOK.1 C2.1 C4.1 C6.1 C8.1 C12.1 C14.1 C21.1 C25.1 C27.1 C29.1 C36.1 C50.1 C54.1 C57.1 CONN3.3 IC1.4 IC4.4 IC5.4 IC7.4 IC8.4 IC9.4 IN_LEFT.4 IN_RIGHT.4 OUT_LEFT.5 OUT_RIGHT.5 R2.1 R31.1 R32.1 R40.1 R43.1 R50.1 R51.1 R63.1 R66.1 TP23.P$1 U4.4 U6.4 U7.4 U8.4
VIO: U$4.VIO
